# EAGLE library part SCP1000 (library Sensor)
Akitsuki Denshi SCP1000 module store WEB site: link
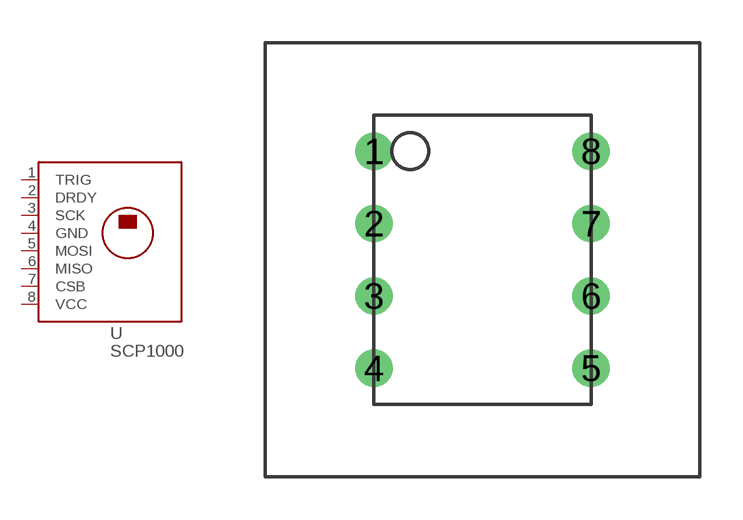
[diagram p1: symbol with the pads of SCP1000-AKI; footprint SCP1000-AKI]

Designator prefix U

## SCP1000AKI  [SCP1000-AKI]
1  TRIG  sup
2  DRDY  sup
3  SCK  in
4  GND  pwr
5  MOSI  in
6  MISO  out
7  CSB  in
8  VCC  pwr

## Footprint SCP1000-AKI (pad centres in mm)
drill 0.8: 1 -3.81,3.81; 2 -3.81,1.27; 3 -3.81,-1.27; 4 -3.81,-3.81; 5 3.81,-3.81; 6 3.81,-1.27; 7 3.81,1.27; 8 3.81,3.81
